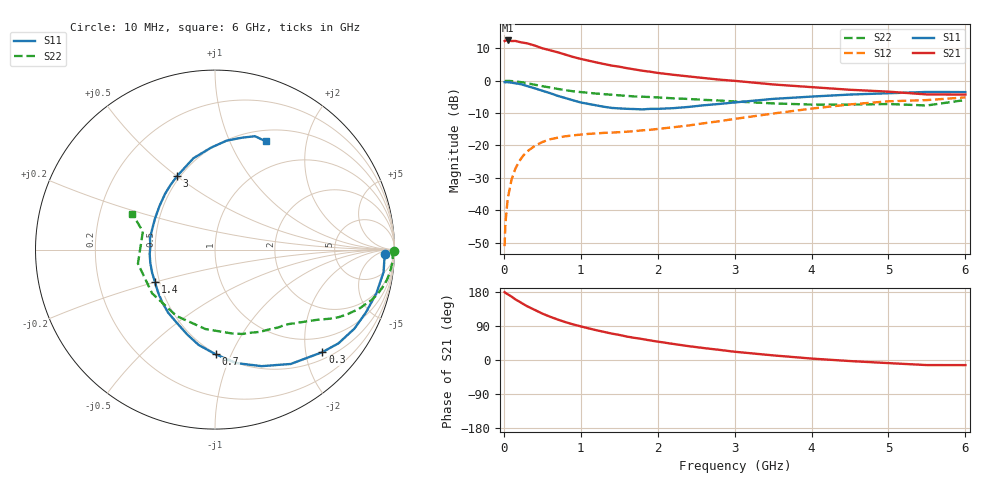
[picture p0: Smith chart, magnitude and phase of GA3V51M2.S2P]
! Infineon Technologies  Discrete & RF Semiconductors
! BF775
! Si NPN RF Bipolar Junction Transistor in SOT23
! VCE = 3.5 V  IC = 1.2 mA
! Common Emitter S-Parameters:  May  1996
# GHz  S  MA  R  50
!  f  S11  S21  S12  S22
! GHz  MAG  ANG  MAG  ANG  MAG  ANG  MAG  ANG
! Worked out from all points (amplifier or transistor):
!   36 points, 10 MHz to 6 GHz, reference 50 ohm
!   highest |S21| = 12.4 dB at 50 MHz (marker M1)
!   |S21| within 3 dB of that: start of sweep to 596.2 MHz
!   unconditionally stable (mu >= 1): 1.37 GHz to 3.944 GHz; 5.14 GHz to end of sweep
!   at 250 MHz: K = 0.21, MSG = 17.4 dB, |S12| = -23.2 dB
!   at 1.4 GHz: K = 1.02, MAG = 9.5 dB, |S12| = -16.0 dB
!   at 6 GHz: K = 1.01, MAG = -0.3 dB, |S12| = -5.2 dB
!   S11 on the Smith chart (normalised r, x): 10 MHz: 30, -14; 300 MHz: 0.65, -2.34; 700 MHz: 0.49, -0.88; 1.4 GHz: 0.47, -0.20; 3 GHz: 0.48, +0.50; 6 GHz: 0.63, +1.37
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0.01  0.9465 -1.5  4.092 179.1  0.0028 90.3  0.9999 -0.6
0.02  0.9452 -3.0  4.165 177.2  0.0062 90.6  0.9868 -1.3
0.05  0.9476 -7.6  4.171 173.6  0.0151 84.1  0.9935 -3.3
0.1  0.9317 -15.2  4.086 167.3  0.0298 81.1  0.9849 -6.6
0.15  0.9103 -22.8  4.102 160.0  0.044 76.0  0.9733 -9.9
0.3  0.8272 -43.7  3.774 142.1  0.0803 64.3  0.9145 -18.0
0.4  0.7641 -56.5  3.487 132.4  0.0983 57.5  0.8668 -22.4
0.5  0.6994 -68.2  3.158 122.5  0.113 52.2  0.8225 -25.9
0.6  0.6428 -79.5  2.945 114.3  0.1246 47.7  0.7845 -28.7
0.7  0.5836 -89.6  2.741 106.8  0.132 44.4  0.7457 -31.1
0.8  0.5392 -99.7  2.525 100.0  0.1386 41.6  0.7136 -33.0
0.9  0.4977 -108.1  2.322 94.0  0.1434 39.6  0.6865 -34.8
1.1  0.4377 -126.6  2.038 83.6  0.151 36.9  0.649 -38.0
1.4  0.3802 -151.8  1.711 69.8  0.1581 35.7  0.6071 -42.6
1.7  0.3648 -176.2  1.49 58.4  0.1663 37.7  0.5705 -47.2
2.2  0.3766 152.6  1.234 42.5  0.191 41.3  0.5346 -56.7
3  0.4612 117.2  0.994 21.8  0.257 43.5  0.4778 -78.2
3.5  0.5234 103.2  0.874 12.2  0.3111 41.1  0.446 -96.7
4.5  0.6107 83.9  0.724 -2.8  0.43 29.7  0.4268 -145.2
5  0.6397 76.8  0.677 -8.2  0.4806 21.8  0.4364 -169.7
5.5  0.67 70.6  0.613 -13.4  0.5017 12.9  0.4143 165.9
6  0.6662 65.0  0.61 -13.5  0.552 8.1  0.5032 156.5
